DATA_BLOCK DB 1
STRUCT
	Value		: INT
	VAR0		: INT
END_STRUCT
BEGIN
	Value		:= 8290
	VAR0		:= 0
END_DATA_BLOCK


FUNCTION_BLOCK FB 1
BEGIN
	__ASSERT==	__AR 2,		P#42.0 // Check AR2 magic

	L		W#16#4321
	T		MW 0
END_FUNCTION_BLOCK


FUNCTION FC 1 : VOID
BEGIN
	__ASSERT==	__AR 2,		P#42.0 // Check AR2 magic

	L		W#16#1234
	T		MW 0
	CALL		FC 2
END_FUNCTION


FUNCTION FC 2 : VOID
BEGIN
	__ASSERT==	__AR 2,		P#42.0 // Check AR2 magic

	L		W#16#6789
	T		MW 0
	L		10
	T		LB 0
END_FUNCTION


FUNCTION FC 3 : VOID
BEGIN
	__ASSERT==	__AR 2,		P#42.0 // Check AR2 magic

	L		1
	T		LB 0
	CALL		FC 2
	__ASSERT==	LB 0,	1
END_FUNCTION


FUNCTION FC 4 : VOID
VAR_INPUT
	INPVAR		: INT
	INPVAR3		: BOOL
	INPVAR4		: BOOL
END_VAR
VAR_IN_OUT
	INOUT0		: INT
	INOUT1		: INT
END_VAR
BEGIN
	__ASSERT==	__AR 2,		P#42.0 // Check AR2 magic

	// Check interface
	L		#INPVAR
	__ASSERT==	__ACCU 1,	9976
	U		#INPVAR3
	__ASSERT==	__STW VKE,	0
	U		#INPVAR4
	__ASSERT==	__STW VKE,	1
	L		#INOUT0
	__ASSERT==	__ACCU 1,	84
	L		#INOUT1
	__ASSERT==	__ACCU 1,	984

	L		42
	T		#INOUT0
	L		942
	T		#INOUT1
END_FUNCTION


FUNCTION FC 5 : VOID
VAR_INPUT
	INPVAR2		: INT
	INPVAR3		: BOOL
	INPVAR4		: BOOL
END_VAR
VAR_IN_OUT
	INOUT0		: INT
	INOUT1		: INT
END_VAR
BEGIN
	__ASSERT==	__AR 2,		P#42.0 // Check AR2 magic

	// Check interface
	L		#INOUT0
	__ASSERT==	__ACCU 1,	84
	L		#INOUT1
	__ASSERT==	__ACCU 1,	984

	CALL FC 4 (
		INPVAR		:= #INPVAR2,	// This is a parameter
		INPVAR3		:= #INPVAR3,
		INPVAR4		:= #INPVAR4,
		INOUT0		:= #INOUT0,
		INOUT1		:= #INOUT1,
	)

	L		#INOUT0
	__ASSERT==	__ACCU 1,	42
	L		168
	T		#INOUT0
	L		#INOUT1
	__ASSERT==	__ACCU 1,	942
	L		9168
	T		#INOUT1
END_FUNCTION


FUNCTION FC 6 : VOID
BEGIN
	__ASSERT==	__AR 2,		P#42.0 // Check AR2 magic

	// Only check OV and OS bits
	__ASSERT==	__STW OV,	1
	__ASSERT==	__STW OS,	0
	L		1
	L		1
	+I
	__ASSERT==	__STW OV,	0
	__ASSERT==	__STW OS,	0
END_FUNCTION


FUNCTION FC 7 : VOID
BEGIN
	__ASSERT==	__AR 2,		P#42.0 // Check AR2 magic

	// Trigger an overflow
	__ASSERT==	__STW OV,	0
	__ASSERT==	__STW OS,	0
	L		30000
	L		30000
	+I
	__ASSERT==	__STW OV,	1
	__ASSERT==	__STW OS,	1
END_FUNCTION


FUNCTION_BLOCK FB 10
VAR_INPUT
	INVAR1		: BOOL
	INVAR2		: BYTE
	INVAR3		: WORD
	INVAR4		: DWORD
	INVAR5		: INT
	INVAR6		: DINT
	INVAR7		: REAL
	INVAR8		: S5TIME
	INVAR9		: TIME
	INVAR10		: DATE
	INVAR11		: CHAR
END_VAR
VAR_OUTPUT
	RETURNVALUE	: INT
END_VAR
BEGIN
	// This FB is CALLed. Check multi instance base register addresse.
	__ASSERT==	__AR 2,		P#DBX 0.0

	// Check parameter values
	U		#INVAR1
	__ASSERT==	__STW VKE,	1
	L		#INVAR2
	__ASSERT==	__ACCU 1,	B#16#12
	L		#INVAR3
	__ASSERT==	__ACCU 1,	W#16#3456
	L		#INVAR4
	__ASSERT==	__ACCU 1,	DW#16#88776655
	L		#INVAR5
	__ASSERT==	__ACCU 1,	8290
	L		#INVAR6
	__ASSERT==	__ACCU 1,	L#999999
	L		#INVAR7
	__ASSERT==	__ACCU 1,	9.876
	L		#INVAR8
	__ASSERT==	__ACCU 1,	S5T#9s
	L		#INVAR9
	__ASSERT==	__ACCU 1,	T#9s
	L		#INVAR10
	__ASSERT==	__ACCU 1,	900
	L		#INVAR11
	__ASSERT==	__ACCU 1,	'c'
	CALL FC 10 (
		INPUTVAR1	:= #INVAR1,
		INPUTVAR2	:= #INVAR2,
		INPUTVAR3	:= #INVAR3,
		INPUTVAR4	:= #INVAR4,
		INPUTVAR5	:= #INVAR5,
		INPUTVAR6	:= #INVAR6,
		INPUTVAR7	:= #INVAR7,
		INPUTVAR8	:= #INVAR8,
		INPUTVAR9	:= #INVAR9,
		INPUTVAR10	:= #INVAR10,
		INPUTVAR11	:= #INVAR11,
		INVAR_DB	:= DB1.DBW 0,
		RET_VAL		:= #RETURNVALUE,
	)

	// AR2 should still be the multi-instance base register, even if it
	// was clobbered in a called FC/FB.
	__ASSERT==	__AR 2,		P#DBX 0.0
END_FUNCTION_BLOCK


DATA_BLOCK DB 10
FB 10
BEGIN
END_DATA_BLOCK


FUNCTION FC 10 : INT
VAR_INPUT
	INPUTVAR1	: BOOL
	INPUTVAR2	: BYTE
	INPUTVAR3	: WORD
	INPUTVAR4	: DWORD
	INPUTVAR5	: INT
	INPUTVAR6	: DINT
	INPUTVAR7	: REAL
	INPUTVAR8	: S5TIME
	INPUTVAR9	: TIME
	INPUTVAR10	: DATE
	INPUTVAR11	: CHAR
	INVAR_DB	: INT
END_VAR
BEGIN
	// This FC is called from an FB. Thus it has the multi-instance base in AR2.
	__ASSERT==	__AR 2,		P#DBX 0.0

	// Check parameter values
	U		#INPUTVAR1
	__ASSERT==	__STW VKE,	1
	L		#INPUTVAR2
	__ASSERT==	__ACCU 1,	B#16#12
	L		#INPUTVAR3
	__ASSERT==	__ACCU 1,	W#16#3456
	L		#INPUTVAR4
	__ASSERT==	__ACCU 1,	DW#16#88776655
	L		#INPUTVAR5
	__ASSERT==	__ACCU 1,	8290
	L		#INPUTVAR6
	__ASSERT==	__ACCU 1,	L#999999
	L		#INPUTVAR7
	__ASSERT==	__ACCU 1,	9.876
	L		#INPUTVAR8
	__ASSERT==	__ACCU 1,	S5T#9s
	L		#INPUTVAR9
	__ASSERT==	__ACCU 1,	T#9s
	L		#INPUTVAR10
	__ASSERT==	__ACCU 1,	900
	L		#INPUTVAR11
	__ASSERT==	__ACCU 1,	'c'

	L		#INVAR_DB
	__ASSERT==	__ACCU 1,	8290


	// Check parameter pointers
	L		P##INPUTVAR1
	UD		DW#16#FFF80000
	__ASSERT==	__ACCU 1,	DW#16#87000000
	L		P##INPUTVAR2
	UD		DW#16#FFF80000
	__ASSERT==	__ACCU 1,	DW#16#87000000
	L		P##INPUTVAR3
	UD		DW#16#FFF80000
	__ASSERT==	__ACCU 1,	DW#16#87000000
	L		P##INPUTVAR4
	UD		DW#16#FFF80000
	__ASSERT==	__ACCU 1,	DW#16#87000000
	L		P##INPUTVAR5
	UD		DW#16#FFF80000
	__ASSERT==	__ACCU 1,	DW#16#87000000
	L		P##INPUTVAR6
	UD		DW#16#FFF80000
	__ASSERT==	__ACCU 1,	DW#16#87000000
	L		P##INPUTVAR7
	UD		DW#16#FFF80000
	__ASSERT==	__ACCU 1,	DW#16#87000000
	L		P##INPUTVAR8
	UD		DW#16#FFF80000
	__ASSERT==	__ACCU 1,	DW#16#87000000
	L		P##INPUTVAR9
	UD		DW#16#FFF80000
	__ASSERT==	__ACCU 1,	DW#16#87000000
	L		P##INPUTVAR10
	UD		DW#16#FFF80000
	__ASSERT==	__ACCU 1,	DW#16#87000000
	L		P##INPUTVAR11
	UD		DW#16#FFF80000
	__ASSERT==	__ACCU 1,	DW#16#87000000


	// Handle and check return value
	L		99
	T		#RET_VAL
	L		#RET_VAL
	__ASSERT==	__ACCU 1,	99
	L		P##RET_VAL
	UD		DW#16#FFF80000
	__ASSERT==	__ACCU 1,	DW#16#87000000


	// And another nested call
	CALL FC 11 (
		IN1	:= #INVAR_DB,
	)

	// Clobber the multi-instance base
	LAR2		P#84.0
END_FUNCTION


FUNCTION FC 11 : VOID
VAR_INPUT
	IN1		: INT
END_VAR
BEGIN
	// This FC is called from an FB via FC. Thus it has the multi-instance base in AR2.
	__ASSERT==	__AR 2,		P#DBX 0.0

	L		#IN1
	__ASSERT==	__ACCU 1,	8290
END_FUNCTION


ORGANIZATION_BLOCK OB 1
BEGIN
	LAR2		P#42.0	// Magic AR2 value


	CALL		FC 1
	__ASSERT==	MW 0,	W#16#6789
	L		0
	T		MW 0
	__ASSERT==	MW 0,	0
	UC		FC 1
	__ASSERT==	MW 0,	W#16#6789
	L		0
	T		MW 0
	__ASSERT==	MW 0,	0
	SET
	CC		FC 1
	__ASSERT==	MW 0,	W#16#6789
	L		0
	T		MW 0
	__ASSERT==	MW 0,	0
	CLR
	CC		FC 1
	__ASSERT==	MW 0,	0

	__ASSERT==	__AR 2,		P#42.0 // Check AR2 magic

	// Test localdata stack
	L		255
	T		LB 0
	__ASSERT==	LB 0,	255
	CALL		FC 3
	__ASSERT==	LB 0,	255

	__ASSERT==	__AR 2,		P#42.0 // Check AR2 magic


	// Test nested FC calls
	L		84
	T		MW 42
	L		984
	T		DB1.DBW 2
	CALL FC 5 (
		INPVAR2		:= 9976,
		INPVAR3		:= FALSE,
		INPVAR4		:= TRUE,
		INOUT0		:= MW 42,
		INOUT1		:= DB1.DBW 2, // DB1.VAR0
	)
	L		MW 42
	__ASSERT==	__ACCU 1,	168
	L		DB1.DBW 2
	__ASSERT==	__ACCU 1,	9168

	__ASSERT==	__AR 2,		P#42.0 // Check AR2 magic


	// Test OV/OS bits over call boundaries
	__STWRST
	L		30000
	L		30000
	+I
	__ASSERT==	__STW OV,	1
	__ASSERT==	__STW OS,	1
	CALL FC 6
	__ASSERT==	__STW OV,	0
	__ASSERT==	__STW OS,	0
	__STWRST
	CALL FC 7
	__ASSERT==	__STW OV,	1
	__ASSERT==	__STW OS,	0

	__ASSERT==	__AR 2,		P#42.0 // Check AR2 magic


	// Test raw FB call
	L		0
	T		MW 0
	CLR
	UC		FB 1
	L		MW 0
	__ASSERT==	__ACCU 1,	W#16#4321
	L		0
	T		MW 0
	SET
	CC		FB 1
	L		MW 0
	__ASSERT==	__ACCU 1,	W#16#4321

	__ASSERT==	__AR 2,		P#42.0 // Check AR2 magic


	// Test indirect calls
	L		0
	T		MW 0
	L		1
	T		MW 50
	CLR
	UC		FC [MW 50]
	L		MW 0
	__ASSERT==	__ACCU 1,	W#16#6789
	L		0
	T		MW 0
	SET
	CC		FC [MW 50]
	L		MW 0
	__ASSERT==	__ACCU 1,	W#16#6789
	L		0
	T		MW 0
	CLR
	UC		FB [MW 50]
	L		MW 0
	__ASSERT==	__ACCU 1,	W#16#4321
	L		0
	T		MW 0
	SET
	CC		FB [MW 50]
	L		MW 0
	__ASSERT==	__ACCU 1,	W#16#4321

	__ASSERT==	__AR 2,		P#42.0 // Check AR2 magic


	// Test parameter forwarding (FB->FC)
	L		900
	T		MW 10
	CALL FB 10, DB 10 (
		INVAR1		:= TRUE,
		INVAR2		:= B#16#12,
		INVAR3		:= W#16#3456,
		INVAR4		:= DW#16#88776655,
		INVAR5		:= DB1.DBW 0,
		INVAR6		:= L#999999,
		INVAR7		:= 9.876,
		INVAR8		:= S5T#9s,
		INVAR9		:= T#9s,
		INVAR10		:= MW 10,
		INVAR11		:= 'c',
		RETURNVALUE	:= MW 0,
	)
	L		MW 0
	__ASSERT==	__ACCU 1,	99

	__ASSERT==	__AR 2,		P#42.0 // Check AR2 magic


	CALL SFC 46 // STOP CPU
END_ORGANIZATION_BLOCK
